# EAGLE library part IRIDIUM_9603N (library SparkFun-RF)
Iridium 9603N Modem Connector is Samtec SS4-10-3.50-L-D-K-TR Requires two HW-14879 M2x0.4 6mm-tall reflow standoffs. The position of the standoffs is shown on the footprint tDocu.
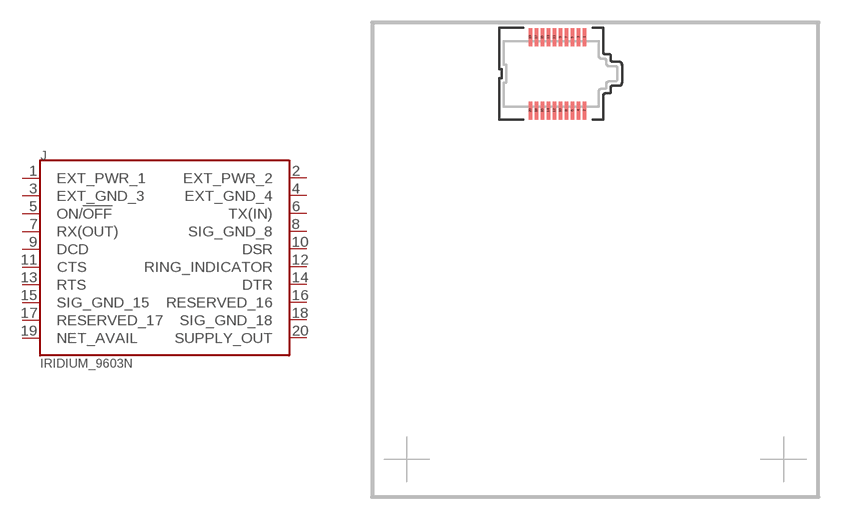
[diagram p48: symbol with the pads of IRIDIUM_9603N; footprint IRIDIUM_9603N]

Designator prefix J

## IRIDIUM_9603N (PROD_ID: CONN-14689; VALUE: IRIDIUM_9603N)  [IRIDIUM_9603N]
1  EXT_PWR_1  pwr
2  EXT_PWR_2  pwr
3  EXT_GND_3  pwr
4  EXT_GND_4  pwr
5  ON/!OFF!  in
6  TX(IN)  in
7  RX(OUT)  out
8  SIG_GND_8  pwr
9  DCD  out
10  DSR  out
11  CTS  out
12  RING_INDICATOR  out
13  RTS  in
14  DTR  in
15  SIG_GND_15  pwr
16  RESERVED_16  nc
17  RESERVED_17  nc
18  SIG_GND_18  pwr
19  NET_AVAIL  out
20  SUPPLY_OUT  out

## Footprint IRIDIUM_9603N (pad centres in mm)
0.4mm[.016] SOCKET STRIP ASSEMBLY.
smd 0.23 x 1.2: 1 1.8,2.435; 2 1.8,-2.435; 3 1.4,2.435; 4 1.4,-2.435; 5 1,2.435; 6 1,-2.435; 7 0.6,2.435; 8 0.6,-2.435; 9 0.2,2.435; 10 0.2,-2.435; 11 -0.2,2.435; 12 -0.2,-2.435; 13 -0.6,2.435; 14 -0.6,-2.435; 15 -1,2.435; 16 -1,-2.435; 17 -1.4,2.435; 18 -1.4,-2.435; 19 -1.8,2.435; 20 -1.8,-2.435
